(* Logix 5000 Rung export; software revision 16.04 *)

MODULES
   Local : vendor None type None code None
   MVI56E_MNET : vendor None type None code None
END_MODULES

TYPE MNETDATA :   // Contains Read Data (data read from the module to the processor) and Write Data (data written from the processor to the module)
STRUCT
   ReadData : INT[600];   // Data read from module. Set array equal to the size set in the Configuration file.
   WriteData : INT[600];   // Data to write to module. Set array equal to the size set in the Configuration file.
END_STRUCT
END_TYPE

TYPE MNETIPADDRESS :   // Data structure to get and set the IP address of the module.
STRUCT
   IPGetTrigger : BOOL;   // Gets IP address.
   IPReceived : INT[4];   // IP address received.
   IPSetTrigger : BOOL;   // Sets IP address
   IPRequested : INT[4];   // IP address set.
END_STRUCT
END_TYPE

TYPE MNETCONTROL :   // Values used by program for data transfer operation between the module and the processor.
STRUCT
   WarmBoot : BOOL;   // Causes software reset. The Module reads new configuration information.
   ColdBoot : BOOL;   // Causes hardware reset.
   BPLastRead : INT;   // Index of last read block
   BPLastWrite : INT;   // Index of last write block
   BlockIndex : INT;   // Computed block offset for data table
   WBPending : BOOL;   // Pending message
   CBPending : BOOL;   // Pending message
   ReadDataBlkCount : INT;   // Holds the value of the Block Counts of the Read Data Array. Array Size is divided by 200.
   WriteDataBlkCount : INT;   // Holds the value of the Block Counts of the Write Data Array. Array Size is divided by 200.
   RBTSremainder : INT;   // Holds remainder calculation value from the read array.
   WBTSremainder : INT;   // Holds remainder calculation value from the write array.
   ReadDataSizeGet : INT;   // Holds read data array size.
   WriteDataSizeGet : INT;   // Holds write data array size.
   IPAddress : MNETIPADDRESS;   // Getting and Setting IP address to and from Module
   FaultCode : INT;   // Fault Code value
   CheckInitialization : BOOL;   // Check Initialization trigger
END_STRUCT
END_TYPE

TYPE MNETEVENTCMD :   // Data structure to use for Event message generation.
STRUCT
   EventCmdTrigger : BOOL;   // Trigger for event command. User ladder must set this bit to initiate event command
   EventCmdPending : BOOL;   // Set after the ladder has sent an event cmd to the module and is waiting for the status to be returned
   IPAddress : INT[4];   // Server IP address. example: 192.168.0.101
   ServicePort : INT;   // TCP Service Port number (0-65535), 502 for MBAP, 2000 for MNET
   SlaveAddress : INT;   // Modbus slave NODE address (0 to 247)
   InternalDBAddress : INT;   // Internal database address
   PointCount : INT;   // Number of points for this command
   SwapCode : INT;   // Swap code (0= no swap, 1=swap words, 2=swap words and bytes, 3=swap bytes)
   ModbusFunctionCode : INT;   // Modbus function code
   DeviceDBAddress : INT;   // Target Server Modbus Address.
   EventCmdStatusReturned : INT;   // (0=Fail, 1=Success)
   EventBlockID : INT;   // Temporary variable to calculate event block ID
END_STRUCT
END_TYPE

TYPE MNETBLKSTAT :   // This object is used to store the block transfer statistics for the MVI56-MNET module.
STRUCT
   Read : INT;   // Total number of read block transfers
   Write : INT;   // Total number of write block transfers
   Parse : INT;   // Total number of blocks parsed
   Event : INT;   // Total number of event blocks received
   Cmd : INT;   // Total number of command blocks received
   Err : INT;   // Total number of block transfer errors
END_STRUCT
END_TYPE

TYPE MNETMODULEDEF :   // This defines the whole module which includes all tags used in the program
STRUCT
   DATA : MNETDATA;   // Data read from module
   STATUS : MNETSTATUS;   // Client ,Server Status and blocks status
   CONTROL : MNETCONTROL;   // MNET Module control warmboot, coldboot, etc
   UTIL : MNETUTIL;   // command, event control
END_STRUCT
END_TYPE

TYPE MNETUTIL :   // Variables for internal ladder usage - should not be accessed by user application
STRUCT
   CmdControl : MNETCMDCONTROL;   // Allows for a disabled command to be sent to a device(Server)
   EventCmd : MNETEVENTCMD;   // Event data to be used
   InitOutputData : MNETINITOUTDATA;   // This is to initialize output data module reads data from PLC
   PassThru : MNETPASSTHRU;   // This is to handle the pass thru format to be passed straight to the processor.
   IPsetPending : BOOL;   // Allows Setting module IP address
   IPgetPending : BOOL;   // Allows Getting module IP address
END_STRUCT
END_TYPE

TYPE MNETCMDCONTROL :   // Controlling the Modbus Commands
STRUCT
   TriggerCmdCntrl : BOOL;   // Trigger Command Control. User application will activate this trigger.
   NumberOfCommands : INT;   // Number of commands per block (1 to 6)
   CommandIndex : INT[6];   // Stores the command indexes for command control.
   CmdsAddedToQueue : INT;   // Number of commands added to queue
   CmdControlBlockID : INT;   // Temporary variable to calculate control block ID
   CmdCntrlPending : BOOL;   // Auxiliary control command - prevents a second request before acknowledgment is received
END_STRUCT
END_TYPE

TYPE MNETSTATUS :   // This status data is returned on each read block and can be used to detect proper module operation.
STRUCT
   PassCnt : INT;   // Program cycle counter
   ProductVersion : INT;   // Shows the module software version
   ProductCode : INT[2];   // This identifies the module product code
   MnetServStats : MNETSTATS;   // Server status for port 502
   MBAPServStats : MNETSTATS;   // Server status for port 2000
   ClientStats : MNETSTATS;   // Client Status
   BlockStats : MNETBLKSTAT;   // Block Transfer Statistics.
END_STRUCT
END_TYPE

TYPE MNETSTATS :   // This object is used to store the port statistics for an MVI56-MNET port.
STRUCT
   CmdReq : INT;   // Total number of command list requests sent
   CmdResp : INT;   // Total number of command list responses received
   CmdErr : INT;   // Total number of command list errors
   Requests : INT;   // Total number of requests for port
   Responses : INT;   // Total number of responses for port
   ErrSent : INT;   // Total number of errors sent
   ErrRec : INT;   // Total number of errors received
   CfgErrWord : INT;   // Configuration Error Word
   CurErr : INT;   // Current Error code
   LastErr : INT;   // Last recorded error code
END_STRUCT
END_TYPE

TYPE MNETPASSTHRU :   // Applicable with the selection of a Pass-Through mode (1 to 3) in the Configuration file.
STRUCT
   MBControl1 : CONTROL;   // Modbus pass thru message control
   MBControl2 : CONTROL;   // Modbus pass thru message control
   Mbdouble : DINT;   // Modbus double int tag
   MBMsg : SINT[500];   // Message array
   MBMsgLen : INT;   // Message length
   MBOffset : INT;   // Start offset in the message
   MBOffsetBit : INT;   // Offset bit in the message
   MBScratch : INT[3];   // Temporary used ints
   MBboolLength : DINT;   // Holds Word size that will accommodate Coil Qty.
   MBSpecial : INT[4];   // Holds Special Function 99 data.
   WriteDataDINTBuffer : DINT[50];   // Hold WriteData in DINT array
   InputDataDINTBuffer : DINT[50];   // Hold Connection Input Data in DINT array
END_STRUCT
END_TYPE

TYPE MNETINITOUTDATA :   // Used to bring the Module into a known state after a restart operation.
STRUCT
   TriggerInitOut : BOOL;   // Trigger Output Data Initialization.
   InitializeOutputData : INT;   // Quantity of Blocks(200 words of "ReadData") for the module to read from the PLC. [0 to 24] means a qty of 1 to 25
   RetInitOutData : INT[200];   // Returned Initialization output data
   TriggerInitOutPending : BOOL;   // Set after the ladder has sent an event cmd to the module and is waiting for the status to be returned
   RetInitOutDataBlkID : INT;   // Returned Block ID for Returned Initialize Output Data command.
   InitOutBlkIDLim : INT;   // Block Index Limit for ReadData size of the array
END_STRUCT
END_TYPE

ADD_ON_INSTRUCTION AOI56MNET   (* revision 1.62, vendor ProSoft Technology Inc., ExecutePrescan *)
// Add-On - MVI56-MNET and  MVI56E-MNET modules.
// Revision note:
// v1.62. resolves minor arithmetic overflow fault when msb of WriteData registers are set during a function 5 or 15 while passthru
VAR_IN_OUT
   Connection_Input : INT[250]; {required}   // Input parameters.
   Connection_Output : INT[248]; {required}   // Output parameters.
   MNET : MNETMODULEDEF; {required}
        .DATA.READDATA[0]   // Reads the RadData array size.
        ._UTIL.PASSTHRU.MBMSG[0]   // Modbus reserved. Always 0.
        ._UTIL.PASSTHRU.MBMSG[3]   // Modbus Function Code received.
        ._UTIL.PASSTHRU.MBOFFSET   // Starting Address for Modbus data set.
END_VAR
VAR
   MJFAULTS : DINT[12];
END_VAR

ROUTINE Logic   (* ladder *)
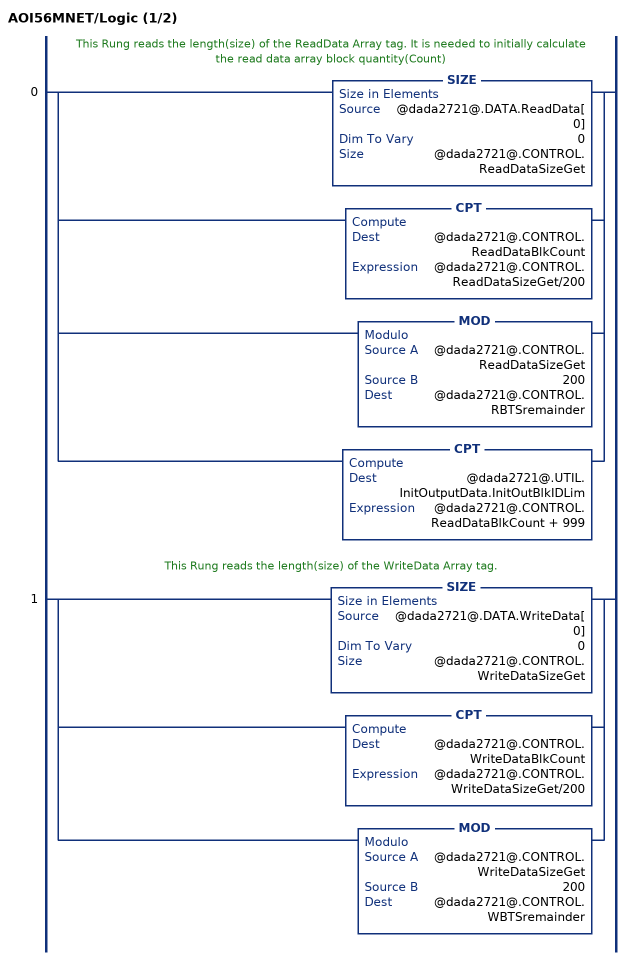
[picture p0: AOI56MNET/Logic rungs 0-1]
   // This Rung reads the length(size) of the ReadData Array tag. It is needed to initially calculate the read data array block quantity(Count)
   0: [SIZE(@dada2721@.DATA.ReadData[0],0,@dada2721@.CONTROL.ReadDataSizeGet) ,CPT(@dada2721@.CONTROL.ReadDataBlkCount,@dada2721@.CONTROL.ReadDataSizeGet/200) ,MOD(@dada2721@.CONTROL.ReadDataSizeGet,200,@dada2721@.CONTROL.RBTSremainder) ,CPT(@dada2721@.UTIL.InitOutputData.InitOutBlkIDLim,@dada2721@.CONTROL.ReadDataBlkCount + 999) ];
   // This Rung reads the length(size) of the WriteData Array tag.
   1: [SIZE(@dada2721@.DATA.WriteData[0],0,@dada2721@.CONTROL.WriteDataSizeGet) ,CPT(@dada2721@.CONTROL.WriteDataBlkCount,@dada2721@.CONTROL.WriteDataSizeGet/200) ,MOD(@dada2721@.CONTROL.WriteDataSizeGet,200,@dada2721@.CONTROL.WBTSremainder) ];
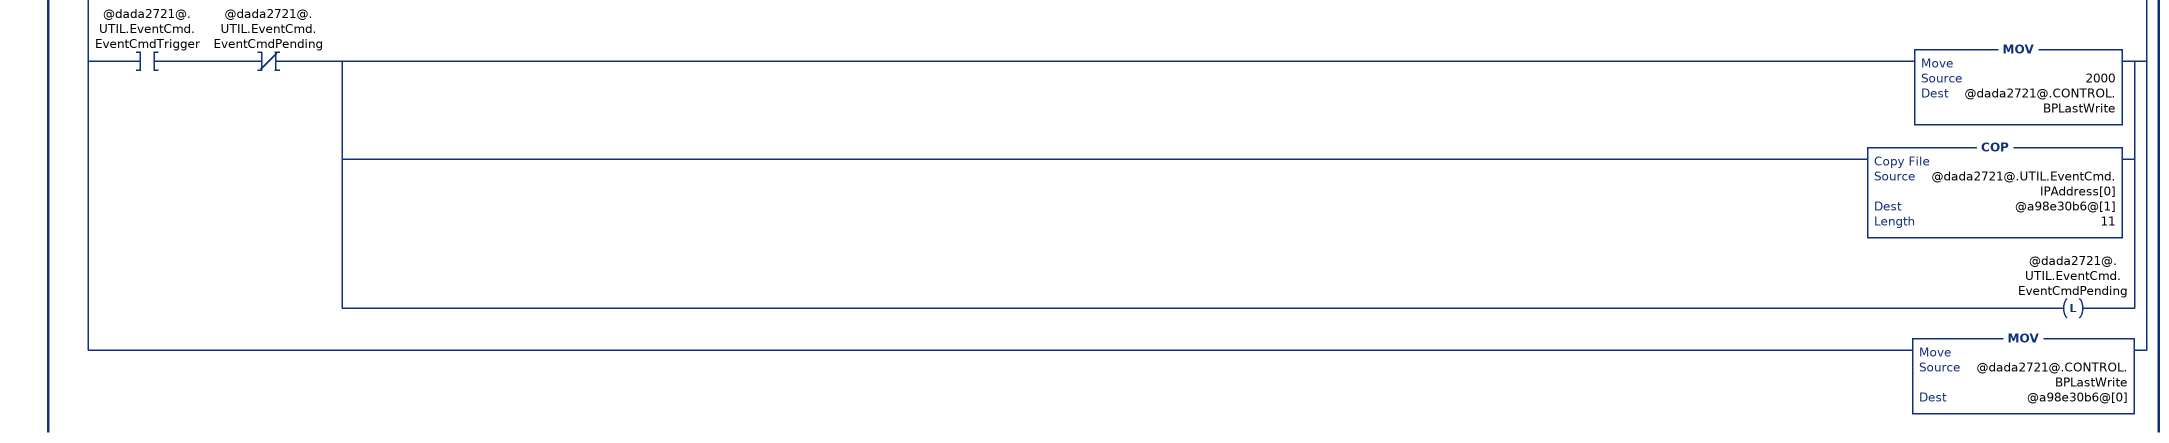
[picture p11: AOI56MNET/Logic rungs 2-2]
   // This rung is used to check for a new read block from the MVI56-MNET module in slot 1.  If new data is available, the LastRead and word[0] will not be equal.  This will force the program to call the ReadData subroutine to process the new data received.  After the new data is placed in the Modbus Data Table, the program will send new data to the module using the WriteData subroutine.
   2: NEQ(@39e2dc0f@[249],@dada2721@.CONTROL.BPLastRead)[MOV(@39e2dc0f@[249],@dada2721@.CONTROL.BPLastRead) ,GRT(@dada2721@.CONTROL.FaultCode,0) OTL(@dada2721@.CONTROL.CheckInitialization) ,EQU(@dada2721@.CONTROL.FaultCode,0) NEQ(@dada2721@.CONTROL.FaultCode,0) OTU(@dada2721@.CONTROL.CheckInitialization) ,EQU(@dada2721@.CONTROL.FaultCode,0) [EQU(-1,@dada2721@.CONTROL.BPLastRead) ,EQU(0,@dada2721@.CONTROL.BPLastRead) ] XIO(@dada2721@.CONTROL.CheckInitialization) [[EQU(@dada2721@.STATUS.ProductCode[1],13637) GEQ(@dada2721@.STATUS.ProductVersion,205) ,EQU(@dada2721@.STATUS.ProductCode[1],13652) GEQ(@dada2721@.STATUS.ProductVersion,151) ] [GEQ(@dada2721@.CONTROL.ReadDataSizeGet,200) COP(@39e2dc0f@[2],@dada2721@.DATA.ReadData[0],200) ,LES(@dada2721@.CONTROL.ReadDataSizeGet,200) COP(@39e2dc0f@[2],@dada2721@.DATA.ReadData[0],@dada2721@.CONTROL.RBTSremainder) ] ,COP(@39e2dc0f@[202],@dada2721@.STATUS.PassCnt,1) ,COP(@39e2dc0f@[203],@dada2721@.STATUS.BlockStats.Read,6) ,COP(@39e2dc0f@[209],@dada2721@.STATUS.ProductCode[0],2) ,COP(@39e2dc0f@[211],@dada2721@.STATUS.ProductVersion,1) ,COP(@39e2dc0f@[219],@dada2721@.STATUS.MnetServStats.CmdReq,10) ,COP(@39e2dc0f@[229],@dada2721@.STATUS.MBAPServStats.CmdReq,10) ,COP(@39e2dc0f@[239],@dada2721@.STATUS.ClientStats.CmdReq,10) ] ,GEQ(@dada2721@.CONTROL.BPLastRead,1) [LEQ(@dada2721@.CONTROL.BPLastRead,@dada2721@.CONTROL.ReadDataBlkCount) [CPT(@dada2721@.CONTROL.BlockIndex,(@dada2721@.CONTROL.BPLastRead-1)*200) ,COP(@39e2dc0f@[2],@dada2721@.DATA.ReadData[@dada2721@.CONTROL.BlockIndex],200) ] ,CMP(@dada2721@.CONTROL.BPLastRead - @dada2721@.CONTROL.ReadDataBlkCount = 1) GRT(@dada2721@.CONTROL.RBTSremainder,0) [CPT(@dada2721@.CONTROL.BlockIndex,(@dada2721@.CONTROL.BPLastRead-1)*200) ,COP(@39e2dc0f@[2],@dada2721@.DATA.ReadData[@dada2721@.CONTROL.BlockIndex],@dada2721@.CONTROL.RBTSremainder) ] ,LEQ(@dada2721@.CONTROL.BPLastRead,25) [MOV(@39e2dc0f@[202],@dada2721@.STATUS.PassCnt) ,COP(@39e2dc0f@[203],@dada2721@.STATUS.BlockStats.Read,6) ,COP(@39e2dc0f@[209],@dada2721@.STATUS.ProductCode[0],2) ,COP(@39e2dc0f@[211],@dada2721@.STATUS.ProductVersion,1) ,COP(@39e2dc0f@[219],@dada2721@.STATUS.MnetServStats.CmdReq,10) ,COP(@39e2dc0f@[229],@dada2721@.STATUS.MBAPServStats.CmdReq,10) ,COP(@39e2dc0f@[239],@dada2721@.STATUS.ClientStats.CmdReq,10) ] ] ,EQU(@dada2721@.CONTROL.BPLastRead,9990) [COP(@39e2dc0f@[2],@dada2721@.CONTROL.IPAddress.IPRequested[0],4) ,OTU(@dada2721@.UTIL.IPsetPending) ] ,EQU(@dada2721@.CONTROL.BPLastRead,9991) [COP(@39e2dc0f@[2],@dada2721@.CONTROL.IPAddress.IPReceived[0],4) ,OTU(@dada2721@.UTIL.IPgetPending) ] ,LIM(9956,@dada2721@.CONTROL.BPLastRead,9996) [EQU(9996,@dada2721@.CONTROL.BPLastRead) [MOV(@39e2dc0f@[2],@dada2721@.UTIL.PassThru.MBMsgLen) ,COP(@39e2dc0f@[3],@dada2721@.UTIL.PassThru.MBMsg[0],@dada2721@.UTIL.PassThru.MBMsgLen) ] ,LIM(9956,@dada2721@.CONTROL.BPLastRead,9957) [MOV(@39e2dc0f@[3],@dada2721@.UTIL.PassThru.MBOffset) ,LES(@dada2721@.UTIL.PassThru.MBOffset,@dada2721@.CONTROL.WriteDataSizeGet) COP(@39e2dc0f@[4],@dada2721@.DATA.WriteData[@dada2721@.UTIL.PassThru.MBOffset],@39e2dc0f@[2]) ] ,EQU(9958,@dada2721@.CONTROL.BPLastRead) [MOV(@39e2dc0f@[3],@dada2721@.UTIL.PassThru.MBOffsetBit) ,MOV(@39e2dc0f@[4],@dada2721@.UTIL.PassThru.MBScratch[2]) ,DIV(@dada2721@.UTIL.PassThru.MBOffsetBit,16,@dada2721@.UTIL.PassThru.MBOffset) ,MOD(@dada2721@.UTIL.PassThru.MBOffsetBit,16,@dada2721@.UTIL.PassThru.MBOffsetBit) ,XPY(2,@dada2721@.UTIL.PassThru.MBOffsetBit,@dada2721@.UTIL.PassThru.mbdouble) ,MVM(@dada2721@.UTIL.PassThru.mbdouble,16#0000_ffff,@dada2721@.UTIL.PassThru.MBOffsetBit) ,COP(@dada2721@.DATA.WriteData[@dada2721@.UTIL.PassThru.MBOffset],@dada2721@.UTIL.PassThru.WriteDataDINTBuffer[0],1) ,GEQ(@dada2721@.UTIL.PassThru.MBOffset,0) LES(@dada2721@.UTIL.PassThru.MBOffset,@dada2721@.CONTROL.WriteDataSizeGet) LEQ(@dada2721@.UTIL.PassThru.MBOffset,2048) [NEQ(@dada2721@.UTIL.PassThru.MBScratch[2],0) OR(@dada2721@.UTIL.PassThru.MBOffsetBit,@dada2721@.DATA.WriteData[@dada2721@.UTIL.PassThru.MBOffset],@dada2721@.UTIL.PassThru.WriteDataDINTBuffer[0]) ,EQU(@dada2721@.UTIL.PassThru.MBScratch[2],0) [NOT(@dada2721@.UTIL.PassThru.MBOffsetBit,@dada2721@.UTIL.PassThru.MBOffsetBit) ,AND(@dada2721@.UTIL.PassThru.MBOffsetBit,@dada2721@.DATA.WriteData[@dada2721@.UTIL.PassThru.MBOffset],@dada2721@.UTIL.PassThru.WriteDataDINTBuffer[0]) ] ,COP(@dada2721@.UTIL.PassThru.WriteDataDINTBuffer[0],@dada2721@.DATA.WriteData[@dada2721@.UTIL.PassThru.MBOffset],1) ] ] ,EQU(9959,@dada2721@.CONTROL.BPLastRead) [[MOV(@39e2dc0f@[3],@dada2721@.UTIL.PassThru.MBOffset) ,CPT(@dada2721@.UTIL.PassThru.MBControl1.LEN,@39e2dc0f@[2]/2+(@39e2dc0f@[2] MOD 2)) MOV(@dada2721@.UTIL.PassThru.MBControl1.LEN,@dada2721@.UTIL.PassThru.MBControl2.LEN) ,CPT(@dada2721@.UTIL.PassThru.MBboolLength,@dada2721@.UTIL.PassThru.MBOffset+@39e2dc0f@[2]) ,COP(@39e2dc0f@[4],@dada2721@.UTIL.PassThru.InputDataDINTBuffer[0],50) ,COP(@dada2721@.DATA.WriteData[@dada2721@.UTIL.PassThru.MBOffset],@dada2721@.UTIL.PassThru.WriteDataDINTBuffer[0],@dada2721@.UTIL.PassThru.MBControl1.LEN) ] ,LEQ(@dada2721@.UTIL.PassThru.MBboolLength,@dada2721@.CONTROL.WriteDataSizeGet) [FAL(@dada2721@.UTIL.PassThru.MBControl1,?,?,ALL,@dada2721@.UTIL.PassThru.WriteDataDINTBuffer[@dada2721@.UTIL.PassThru.MBControl1.POS],@dada2721@.UTIL.PassThru.WriteDataDINTBuffer[@dada2721@.UTIL.PassThru.MBControl1.POS] AND(NOT @dada2721@.UTIL.PassThru.InputDataDINTBuffer[25+@dada2721@.UTIL.PassThru.MBControl1.POS])) ,FAL(@dada2721@.UTIL.PassThru.MBControl2,?,?,ALL,@dada2721@.UTIL.PassThru.WriteDataDINTBuffer[@dada2721@.UTIL.PassThru.MBControl2.POS],@dada2721@.UTIL.PassThru.WriteDataDINTBuffer[@dada2721@.UTIL.PassThru.MBControl2.POS] OR(@dada2721@.UTIL.PassThru.InputDataDINTBuffer[25+@dada2721@.UTIL.PassThru.MBControl2.POS] AND @dada2721@.UTIL.PassThru.InputDataDINTBuffer[@dada2721@.UTIL.PassThru.MBControl2.POS])) ,RES(@dada2721@.UTIL.PassThru.MBControl1) ,RES(@dada2721@.UTIL.PassThru.MBControl2) ,COP(@dada2721@.UTIL.PassThru.WriteDataDINTBuffer[0],@dada2721@.DATA.WriteData[@dada2721@.UTIL.PassThru.MBOffset],@39e2dc0f@[2]) ] ] ,LIM(9960,@dada2721@.CONTROL.BPLastRead,9961) [MOV(@39e2dc0f@[3],@dada2721@.UTIL.PassThru.MBOffset) ,MOV(@39e2dc0f@[2],@dada2721@.UTIL.PassThru.MBMsgLen) ,COP(@39e2dc0f@[4],@dada2721@.DATA.WriteData[@dada2721@.UTIL.PassThru.MBOffset],@dada2721@.UTIL.PassThru.MBMsgLen) ,CPT(@dada2721@.UTIL.PassThru.MBMsgLen,@dada2721@.UTIL.PassThru.MBMsgLen*2+2) ,COP(@39e2dc0f@[3],@dada2721@.UTIL.PassThru.MBMsg[0],@dada2721@.UTIL.PassThru.MBMsgLen) ] ,EQU(9970,@dada2721@.CONTROL.BPLastRead) COP(@a98e30b6@[0],@dada2721@.UTIL.PassThru.MBSpecial[0],4) ] ,LIM(5001,@dada2721@.CONTROL.BPLastRead,5006) [MOV(@dada2721@.CONTROL.BPLastRead,@dada2721@.UTIL.CmdControl.CmdControlBlockID) ,MOV(@39e2dc0f@[2],@dada2721@.UTIL.CmdControl.CmdsAddedToQueue) ,OTU(@dada2721@.UTIL.CmdControl.CmdCntrlPending) ,OTU(@dada2721@.UTIL.CmdControl.TriggerCmdCntrl) ] ,EQU(@dada2721@.CONTROL.BPLastRead,2000) [MOV(@dada2721@.CONTROL.BPLastRead,@dada2721@.UTIL.EventCmd.EventBlockID) ,MOV(@39e2dc0f@[2],@dada2721@.UTIL.EventCmd.EventCmdStatusReturned) ,OTU(@dada2721@.UTIL.EventCmd.EventCmdPending) ,OTU(@dada2721@.UTIL.EventCmd.EventCmdTrigger) ] ,MOV(@39e2dc0f@[1],@dada2721@.CONTROL.BPLastWrite) ,XIC(@dada2721@.CONTROL.WarmBoot) [MOV(9998,@dada2721@.CONTROL.BPLastWrite) ,OTU(@dada2721@.CONTROL.WarmBoot) ] ,XIC(@dada2721@.CONTROL.ColdBoot) [MOV(9999,@dada2721@.CONTROL.BPLastWrite) ,OTU(@dada2721@.CONTROL.ColdBoot) ] ,[EQU(-1,@dada2721@.CONTROL.BPLastWrite) ,EQU(0,@dada2721@.CONTROL.BPLastWrite) ] [EQU(@dada2721@.STATUS.ProductCode[1],13637) GEQ(@dada2721@.STATUS.ProductVersion,205) ,EQU(@dada2721@.STATUS.ProductCode[1],13652) GEQ(@dada2721@.STATUS.ProductVersion,151) ] [GEQ(@dada2721@.CONTROL.WriteDataSizeGet,200) COP(@dada2721@.DATA.WriteData[0],@a98e30b6@[1],200) ,LES(@dada2721@.CONTROL.WriteDataSizeGet,200) COP(@dada2721@.DATA.WriteData[0],@a98e30b6@[1],@dada2721@.CONTROL.WBTSremainder) ] ,GEQ(@dada2721@.CONTROL.BPLastWrite,1) [LEQ(@dada2721@.CONTROL.BPLastWrite,@dada2721@.CONTROL.WriteDataBlkCount) [CPT(@dada2721@.CONTROL.BlockIndex,(@dada2721@.CONTROL.BPLastWrite-1)*200) ,COP(@dada2721@.DATA.WriteData[@dada2721@.CONTROL.BlockIndex],@a98e30b6@[1],200) ] ,CMP(@dada2721@.CONTROL.BPLastWrite - @dada2721@.CONTROL.WriteDataBlkCount = 1) GRT(@dada2721@.CONTROL.WBTSremainder,0) [CPT(@dada2721@.CONTROL.BlockIndex,(@dada2721@.CONTROL.BPLastWrite-1)*200) ,COP(@dada2721@.DATA.WriteData[@dada2721@.CONTROL.BlockIndex],@a98e30b6@[1],@dada2721@.CONTROL.WBTSremainder) ] ] ,LIM(1000,@dada2721@.CONTROL.BPLastWrite,1024) LEQ(@dada2721@.CONTROL.BPLastWrite,@dada2721@.UTIL.InitOutputData.InitOutBlkIDLim) [CPT(@dada2721@.CONTROL.BlockIndex,(@dada2721@.CONTROL.BPLastWrite-1000)*200) ,COP(@dada2721@.DATA.ReadData[@dada2721@.CONTROL.BlockIndex],@a98e30b6@[1],200) ] ,XIC(@dada2721@.CONTROL.IPAddress.IPSetTrigger) XIO(@dada2721@.UTIL.IPsetPending) [COP(@dada2721@.CONTROL.IPAddress.IPRequested[0],@a98e30b6@[1],4) ,MOV(9990,@dada2721@.CONTROL.BPLastWrite) ,OTU(@dada2721@.CONTROL.IPAddress.IPSetTrigger) ,OTL(@dada2721@.UTIL.IPsetPending) ] ,XIC(@dada2721@.CONTROL.IPAddress.IPGetTrigger) XIO(@dada2721@.UTIL.IPgetPending) [MOV(9991,@dada2721@.CONTROL.BPLastWrite) ,OTU(@dada2721@.CONTROL.IPAddress.IPGetTrigger) ,OTL(@dada2721@.UTIL.IPgetPending) ] ,XIC(@dada2721@.UTIL.CmdControl.TriggerCmdCntrl) XIO(@dada2721@.UTIL.CmdControl.CmdCntrlPending) [COP(@dada2721@.UTIL.CmdControl.CommandIndex[0],@a98e30b6@[1],6) ,LIM(1,@dada2721@.UTIL.CmdControl.NumberOfCommands,6) ADD(5000,@dada2721@.UTIL.CmdControl.NumberOfCommands,@dada2721@.CONTROL.BPLastWrite) ,OTL(@dada2721@.UTIL.CmdControl.CmdCntrlPending) ] ,XIC(@dada2721@.UTIL.EventCmd.EventCmdTrigger) XIO(@dada2721@.UTIL.EventCmd.EventCmdPending) [MOV(2000,@dada2721@.CONTROL.BPLastWrite) ,COP(@dada2721@.UTIL.EventCmd.IPAddress[0],@a98e30b6@[1],11) ,OTL(@dada2721@.UTIL.EventCmd.EventCmdPending) ] ,MOV(@dada2721@.CONTROL.BPLastWrite,@a98e30b6@[0]) ];
END_ROUTINE

ROUTINE Prescan   (* ladder *)
// Startup
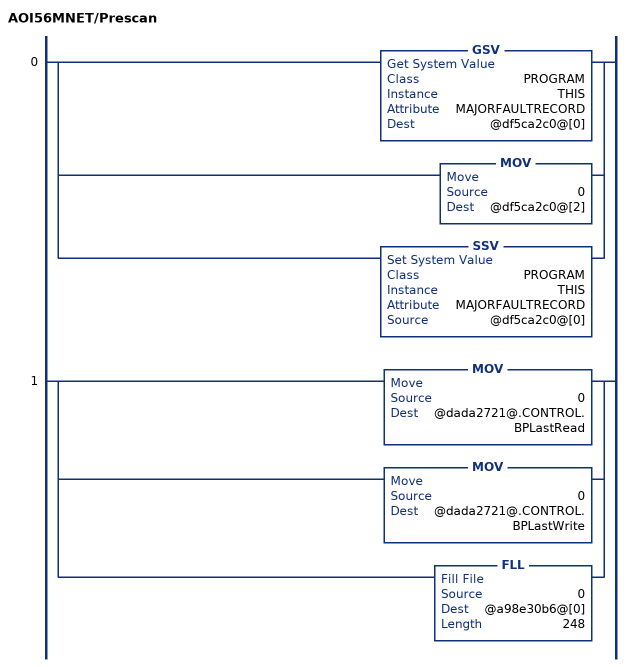
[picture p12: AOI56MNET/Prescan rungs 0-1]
   0: [GSV(PROGRAM,THIS,MAJORFAULTRECORD,@df5ca2c0@[0]) ,MOV(0,@df5ca2c0@[2]) ,SSV(PROGRAM,THIS,MAJORFAULTRECORD,@df5ca2c0@[0]) ];
   1: [MOV(0,@dada2721@.CONTROL.BPLastRead) ,MOV(0,@dada2721@.CONTROL.BPLastWrite) ,FLL(0,@a98e30b6@[0],248) ];
END_ROUTINE
END_ADD_ON_INSTRUCTION

VAR_GLOBAL   (* controller tags *)
   Local:1:I : AB:1756_MODULE_INT_500Bytes:I:0;
   Local:1:O : AB:1756_MODULE_INT_496Bytes:O:0;
   MNET : MNETMODULEDEF;   // Output parameters.
        .DATA.READDATA[0]   // Reads the ReadData array size.
        ._UTIL.PASSTHRU.MBMSG[0]   // Modbus reserved. Always 0.
        ._UTIL.PASSTHRU.MBMSG[3]   // Modbus Function Code received.
        ._UTIL.PASSTHRU.MBOFFSET   // Starting Address for Modbus data set.
   AOI56MNET : AOI56MNET;
END_VAR

PROGRAM MainProgram

ROUTINE MainRoutine   (* ladder *)
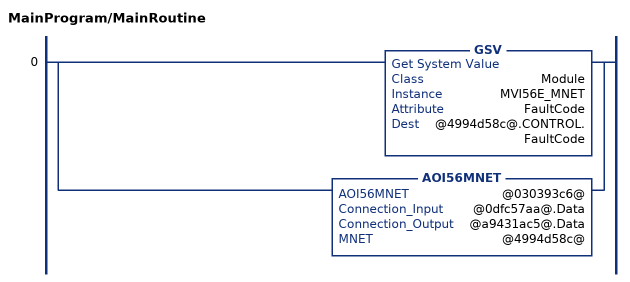
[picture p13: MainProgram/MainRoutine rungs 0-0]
   0: [GSV(Module,MVI56E_MNET,FaultCode,@4994d58c@.CONTROL.FaultCode) ,AOI56MNET(@030393c6@,@0dfc57aa@.Data,@a9431ac5@.Data,@4994d58c@) ];
END_ROUTINE
END_PROGRAM
